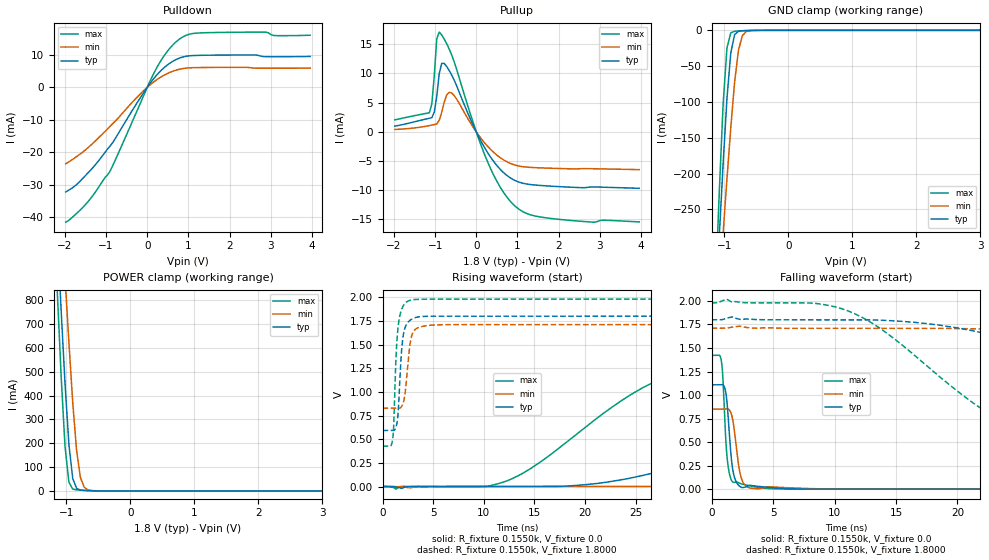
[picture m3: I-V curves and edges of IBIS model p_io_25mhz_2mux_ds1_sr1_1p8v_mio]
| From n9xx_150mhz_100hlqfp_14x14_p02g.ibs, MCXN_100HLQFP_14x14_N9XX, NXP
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[Model] p_io_25mhz_2mux_ds1_sr1_1p8v_mio
|   Model p_io_25mhz_2mux_ds1_sr1_1p8v_mio
| This model was characterised for following simulation conditions:
| External (pad) voltage:
|   - Typ: 1.8V,   - Min: 1.71V,   - Max: 1.98V
| Library cells for typ/min/max conditions are connected as defined below:
|  pad - External Pad
|  ipp_do_lv - Core Input
|  ipp_obe_lv - Output Buffer Enable
|  IOGC - NC
|  REFH3V3 - REFH3V3
|  REFL3V3 - REFL3V3
|  ZI - NC
|  abut_ncal_vddio[1] - vssio vddio vddio
|  abut_ncal_vddio[2] - vddio vddio vssio
|  abut_ncal_vddio[3] - vddio
|  abut_ncal_vddio[4] - vssio vddio vddio
|  abut_ncal_vddio[5] - vddio vddio vssio
|  abut_ncal_vddio[6] - vddio
|  abut_pcal_vddio[1] - vssio
|  abut_pcal_vddio[2] - vddio vssio vddio
|  abut_pcal_vddio[3] - vssio
|  abut_pcal_vddio[4] - vssio
|  abut_pcal_vddio[5] - vddio vssio vddio
|  abut_pcal_vddio[6] - vssio
|  ipp_do_1p8v - ipp_do_1p8v
|  ipp_dse_lv - vdd_lv
|  ipp_eftd_lv - NC
|  ipp_ina_mux_vddio - NC
|  ipp_ina_mux_vddio[0] - NC
|  ipp_ina_mux_vddio[1] - NC
|  ipp_ina_r0_vddio - NC
|  ipp_ina_r0a_vddio - NC
|  ipp_ina_r0b_vddio - NC
|  ipp_ina_r0c_vddio - NC
|  ipp_ina_r0d_vddio - NC
|  ipp_ina_r0e_vddio - NC
|  ipp_ina_r0f_vddio - NC
|  ipp_ina_r300_vddio - NC
|  ipp_ina_r300a_vddio - NC
|  ipp_ina_r300b_vddio - NC
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Model_type I/O
Polarity   Non-Inverting
Enable   Active-High
Vinl =   0.5400V
Vinh =   1.2600V
Vmeas =  0.9000V
Cref =   30.0000pF
Rref =   1.0000M
Vref =   1.8000V
C_comp   1.3067pF   1.2540pF   1.3694pF
|C_comp_pullup   0.5685pF   0.5977pF   0.5417pF
|C_comp_pulldown   0.6639pF   0.6956pF   0.6390pF
[Model Spec]
| variable   typ   min   max
Vinh   1.2600V   1.1970V   1.3860V
Vinl   0.5400V   0.5130V   0.5940V
[Temperature Range]   25.0000   0.1250k   -40.0000
[Voltage Range]   1.8000V   1.7100V   1.9800V
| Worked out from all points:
|   slope of the pulldown table from 0 to 0.27 V, typ, clamps not added: 62.4 ohm
|   slope of the pullup table from 0 to 0.27 V, typ, clamps not added: 77.5 ohm
|   GND clamp passes 1 mA (typ) near -0.75 V on its own axis
|   POWER clamp passes 1 mA (typ) near -0.63 V on its own axis
|   rising waveform, R_fixture 0.1550k, V_fixture 0.0: 20-80 % time 23.2ns typ, 43.7ns min, 11.7ns max; typ from 0 V to 1.11 V
|   rising waveform, R_fixture 0.1550k, V_fixture 1.8000: 20-80 % time 420ps typ, 510ps min, 382ps max; typ from 0.592 V to 1.8 V
|   falling waveform, R_fixture 0.1550k, V_fixture 0.0: 20-80 % time 425ps typ, 524ps min, 366ps max; typ from 1.11 V to 0 V
|   falling waveform, R_fixture 0.1550k, V_fixture 1.8000: 20-80 % time 18.9ns typ, 36.9ns min, 9.36ns max; typ from 1.8 V to 0.592 V
[Pulldown]
|Voltage   I(typ)   I(min)   I(max)
-1.98V    -32.19mA   -23.51mA   -41.49mA
-1.74V    -30.15mA   -21.53mA   -39.06mA
-1.44V    -26.34mA   -18.56mA   -35.19mA
-900mV    -18.01mA   -11.95mA   -25.73mA
180mV     3.037mA    1.878mA    4.81mA
480mV     6.798mA    4.207mA    10.95mA
780mV     8.998mA    5.569mA    14.83mA
1.02V     9.703mA    6.009mA    16.35mA
1.38V     9.882mA    6.118mA    16.81mA
2.88V     9.44mA     5.884mA    17mA
3.12V     9.433mA    5.887mA    15.93mA
3.96V     9.527mA    5.94mA     16.05mA
[Pullup]
|Voltage   I(typ)   I(min)   I(max)
-1.98V    966.3uA    399.3uA    2.044mA
-1.14V    2.321mA    1.063mA    3.243mA
-1.08V    2.416mA    1.15mA     4.764mA
-1.02V    3.358mA    1.24mA     9.557mA
-960mV    6.04mA     1.332mA    15.9mA
-900mV    9.92mA     1.974mA    17.06mA
-780mV    11.71mA    5.034mA    15.89mA
-600mV    9.758mA    6.666mA    13.21mA
240mV     -3.146mA   -2.189mA   -4.533mA
900mV     -8.184mA   -5.592mA   -12.42mA
1.68V     -9.239mA   -6.201mA   -14.7mA
3.96V     -9.667mA   -6.471mA   -15.41mA
[GND_clamp]
|Voltage   I(typ)   I(min)   I(max)
-1.98V    -2A        -1.65A     -2.499A
-1.14V    -394mA     -441.5mA   -363.8mA
-1.08V    -288.3mA   -361.7mA   -226.5mA
-1.02V    -187.2mA   -283.6mA   -103.8mA
-960mV    -95.65mA   -208mA     -24.73mA
-900mV    -31.48mA   -136.2mA   -3.446mA
-840mV    -6.013mA   -72.18mA   -1.335mA
-780mV    -1.302mA   -27.91mA   -907.3uA
-720mV    -579.6uA   -7.636mA   -620.4uA
-660mV    -347.7uA   -1.81mA    -390uA
-420mV    -12.74uA   -30.28uA   -7.287uA
3.96V     0A         0A         0A
[POWER_clamp]
|Voltage   I(typ)   I(min)   I(max)
-1.98V    5.618A     5.349A     6.084A
-1.14V    1.071A     1.443A     829.6mA
-1.08V    754.2mA    1.168A     476.4mA
-1.02V    449mA      895.6mA    184.6mA
-960mV    195.8mA    625.5mA    36.76mA
-900mV    52.43mA    371.1mA    7.779mA
-840mV    10.73mA    170.2mA    4.41mA
-780mV    3.609mA    56.22mA    3.161mA
-720mV    2.066mA    15.04mA    2.177mA
-660mV    1.299mA    4.297mA    1.362mA
-360mV    4.834uA    27.3uA     1.2uA
3.96V     0A         0A         0A
[Ramp]
| variable   typ   min   max
dV/dt_r  0.6652/23.1895n   0.5082/43.6924n   0.8531/11.7283n
dV/dt_f  0.7249/18.8593n   0.5286/36.9351n   0.9321/9.3584n
R_load = 0.1550k
[Rising Waveform]
R_fixture= 0.1550k
V_fixture= 0.0
V_fixture_min= 0.0
V_fixture_max= 0.0
|time   V(typ)   V(min)   V(max)
0s        408.8pV    135.5nV    11.61pV
11.76ns   -24.19uV   -7.747uV   40.52mV
26.88ns   146.7mV    1.659mV    1.105V
32.6ns    317.1mV    17.77mV    1.263V
41.47ns   615.6mV    79.1mV     1.349V
49.41ns   830mV      166.1mV    1.383V
60.71ns   971.3mV    318.1mV    1.404V
83.28ns   1.063V     603.4mV    1.418V
102.6ns   1.089V     722.9mV    1.421V
235ns     1.109V     847mV      1.422V
[Rising Waveform]
R_fixture= 0.1550k
V_fixture= 1.8000
V_fixture_min= 1.7100
V_fixture_max= 1.9800
|time   V(typ)   V(min)   V(max)
0s        591.8mV    826.8mV    426.5mV
1.007ns   591.5mV    826.9mV    506.3mV
1.102ns   591.9mV    826.9mV    642.5mV
1.388ns   652.1mV    826.8mV    1.489V
1.72ns    1.147V     829.4mV    1.81V
1.924ns   1.492V     852.6mV    1.881V
2.149ns   1.652V     931.2mV    1.926V
2.749ns   1.759V     1.529V     1.968V
3.281ns   1.786V     1.664V     1.976V
235ns     1.8V       1.71V      1.98V
[Falling Waveform]
R_fixture= 0.1550k
V_fixture= 0.0
V_fixture_min= 0.0
V_fixture_max= 0.0
|time   V(typ)   V(min)   V(max)
0s        1.109V     850.6mV    1.422V
796.7ps   1.11V      850.5mV    1.361V
906.8ps   1.111V     850.5mV    1.211V
1.241ns   943.7mV    853.6mV    367.1mV
1.606ns   328.6mV    799.6mV    97.7mV
1.94ns    95.78mV    528.4mV    76.01mV
2.258ns   33.84mV    208.7mV    64.31mV
2.586ns   18.09mV    66.15mV    51.62mV
4.885ns   16.12mV    24.46mV    4.902mV
235ns     91.31nV    1.851uV    12.17nV
[Falling Waveform]
R_fixture= 0.1550k
V_fixture= 1.8000
V_fixture_min= 1.7100
V_fixture_max= 1.9800
|time   V(typ)   V(min)   V(max)
0s        1.8V       1.71V      1.98V
10.62ns   1.8V       1.71V      1.917V
13.95ns   1.795V     1.71V      1.687V
23.72ns   1.611V     1.696V     723mV
35.62ns   1.114V     1.597V     499.8mV
42.61ns   865.4mV    1.501V     468mV
50.59ns   744.5mV    1.368V     449.7mV
67.77ns   652.7mV    1.091V     433.8mV
88.47ns   615.7mV    947mV      428.4mV
235ns     591.8mV    829mV      426.5mV
